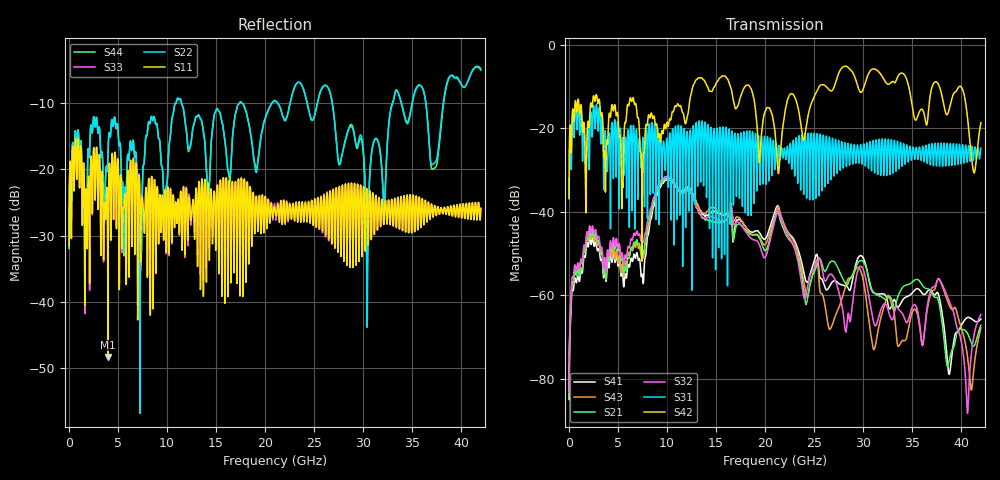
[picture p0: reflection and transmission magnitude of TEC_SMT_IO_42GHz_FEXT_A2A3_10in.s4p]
!! CHANNEL DESCRIPTION: Next Generation 28Gbps High Density SMT I/O Connector
!!  with 10" 5-6-5 Megatron 6 Stripline trace on host side and 1.25" 7-5-7 Megtron 6 Microstrip trace on plug side at 14GHz
!! HOST PCB DESCRIPTION: PCB thickness 2.86 mm, Nelco 4000-13SI (Dk 3.32, Df 0.010)
!!  23 Layer Board, 12 GND planes, 2 Layer route-out on Layers 10,12, 8 mil stub on vias
!!  Pairs on following layers
!!  Layer 10 - A2A3
!! CONNECTOR DESCRIPTION:  Next Generation 28Gbps High Density SMT I/O Connector
!! PLUG-IN CARD DESCRIPTION:  PCB thickness 1mm thick, Nelco 4000-13SI (Dk 3.32, Df 0.010)
!!  6 Layer Board, 4 GND planes, 0.35 x 1.4mm mating pads
!!  Micro-strip diff traces referenced to GND plane 3mils down, 2nd GND plane 15mils from top of board
!!  PCB GND planes are symmetric
!! MODEL DESCRIPTION: TE Connectivity S-parameter model produced from Macro-model
!! MODEL DATE: 9/25/2014 CR1a_GC1i, VR6&12_4
!! MODEL STATUS: Developmental
!! MODEL GEOMETRY: 2 Rows - Rows A, B. 3 pairs in each row, 6 total pairs
!! MODEL FREQUENCY RANGE: DC to 42 GHz in 10 MHz frequency steps
!! MODEL EDGE RATE LIMITATION: 11.90 ps (Using conservative 0.5/Fmax rule of thumb)
!! TIME-DOMAIN TRANSFORM CAUTIONS:
!! 1.) Do not simulate transient edge rates faster than the number listed above.  Edge
!!  rates faster than this number contain significant spectral content at frequencies
!!  above the model's highest frequency.
!! 2.) Even when simulating edge rates that are slower than the number listed above, be
!!  aware that the best time resolution possible with a direct iFFT is (1 / 2Fmax).
!!  As a result, time resolution is typically not adequate for most time-domain
!!  simulations unless tricks such as frequency-domain zero-padding and windowing are
!!  used to minimize leakage and aliasing.
!! 3.) Because the model has a uniform frequency step, a direct iFFT will result in an
!!  impulse that that has a time length given by either (1 / Fstep) or (1 / 2Fstep),
!!  depending on the transform being used.  Care has been taken in selecting the
!!  frequency step to ensure a settled impulse response for the model.  Therefore,
!!  convolution with the model's impulse response should present no issues.  However,
!!  if directly concatenating s-parameter models in the frequency domain a user must
!!  either interpolate necessary interim frequencies or complete impulse response
!!  zero-padding.  Impulse response zero-padding is more difficult, but more accurate.
!! PORT DEFINITIONS:
!! Port  1  ----->  Host, Bot Row  A2  B5  Module, Top Row  <-----  Port  2
!! Port  3  ----->  Host, Bot Row  A3  B6  Module, Top Row  <-----  Port  4
# Hz S MA R 50
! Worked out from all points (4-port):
!   4200 points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, 10 MHz to 42 GHz, reference 50 ohm
!   strongest paths, dB at 10 MHz, 10.51 GHz, 21.01 GHz, 31.51 GHz, 42 GHz:
!     S42: -36.7, -16.2, -21.0, -6.3, -18.7
!     S31: -37.0, -22.1, -28.8, -28.5, -24.8
!     S32: -83.4, -32.5, -41.9, -65.7, -64.6
!     S21: -84.1, -32.9, -41.3, -60.0, -67.2
!     S43: -84.2, -32.4, -41.0, -68.4, -67.9
!     S41: -85.0, -32.9, -39.8, -59.7, -65.7
!   lowest |S11| = -48.3 dB at 3.97 GHz (marker M1), VSWR 1.01, Z = 50.2 + j0.299 ohm
!   |S11| at or under -10 dB: start of sweep to end of sweep
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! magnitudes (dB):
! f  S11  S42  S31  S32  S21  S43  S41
! 10 MHz  -31.6  -36.7  -37.0  -83.4  -84.1  -84.2  -85.0
! 1.95 GHz  -21.5  -18.3  -19.9  -45.9  -46.8  -47.0  -48.4
! 3.97 GHz  -48.3  -22.2  -26.2  -49.4  -51.0  -49.8  -51.9
! 10.21 GHz  -32.5  -18.3  -23.5  -31.8  -32.3  -31.9  -32.4
! 26.2 GHz  -28.5  -10.0  -22.6  -56.5  -54.0  -63.9  -58.6
! 30.42 GHz  -24.6  -7.7  -24.1  -58.1  -54.4  -63.2  -54.4
! 42 GHz  -25.9  -18.7  -24.8  -64.6  -67.2  -67.9  -65.7
